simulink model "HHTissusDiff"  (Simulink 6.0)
settings: Solver=ode45  StartTime=0.0  StopTime=100  RelTol=1e-3
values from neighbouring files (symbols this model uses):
  b = S/Sm    (= 0.1)    [Constantes.m]    (also in ConstantesBck.m)
  C = 1    [Constantes.m]    (also in ConstantesBck.m)
  gk = 36    [Constantes.m]    (also in ConstantesBck.m; sim_hh.m)
  gl = 0.3    [Constantes.m]    (also in ConstantesBck.m; sim_hh.m)
  gna = 120    [Constantes.m]    (also in ConstantesBck.m; sim_hh.m)
  h0 = 0.5961    [Constantes.m]    (also in ConstantesBck.m)
  m0 = 0.0529    [Constantes.m]    (also in ConstantesBck.m)
  mK = 0    [Constantes.m]    (also in ConstantesBck.m)
  mL = 0    [Constantes.m]    (also in ConstantesBck.m)
  mNa = 0    [Constantes.m]    (also in ConstantesBck.m)
  n0 = 0.3177    [Constantes.m]    (also in ConstantesBck.m)
  Rext = 2.9E3    (= 2900)    [Constantes.m]    (also in ConstantesBck.m)
  Rint = 2.9E2    (= 290)    [Constantes.m]    (also in ConstantesBck.m = 400)
  Sm = 3.14e-2    (= 0.0314)    [Constantes.m]    (also in ConstantesBck.m = 0.000314)
  Vdd = 3.3*Rcan/Rct*1000    (= 3.2147881681)    [Constantes.m]    (also in ConstantesBck.m = 1.8)
  Vk = -82    [Constantes.m]    (also in ConstantesBck.m)
  Vl = -59    [Constantes.m]    (also in ConstantesBck.m)
  Vna = 45    [Constantes.m]    (also in ConstantesBck.m)
  Vr = -70    [Constantes.m]    (also in ConstantesBck.m)
libraries: simulink x2

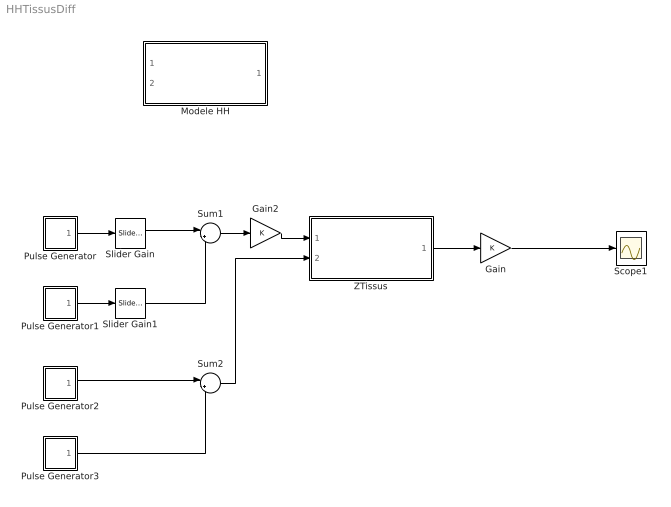
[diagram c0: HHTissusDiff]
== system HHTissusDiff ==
  Gain : Gain
  Gain2 : Gain
  Modele HH : Subsystem
  Pulse Generator : Subsystem  mask(Pulse Generator){period=50, duty=4, amplitude=-1E-2, start=10}
      mask prompts: period "Period (secs):"; duty "Duty cycle (% of period):"; start "Start time:"
      mask help: Pulse Generator
  Pulse Generator1 : Subsystem  mask(Pulse Generator){period=50, duty=4, amplitude=1E-2, start=12}
      mask prompts: period "Period (secs):"; duty "Duty cycle (% of period):"; start "Start time:"
      mask help: Pulse Generator
  Pulse Generator2 : Subsystem  mask(Pulse Generator){period=50, duty=4, amplitude=Vdd, start=10}
      mask prompts: period "Period (secs):"; duty "Duty cycle (% of period):"; start "Start time:"
      mask help: Pulse Generator
  Pulse Generator3 : Subsystem  mask(Pulse Generator){period=50, duty=4, amplitude=-Vdd, start=14}
      mask prompts: period "Period (secs):"; duty "Duty cycle (% of period):"; start "Start time:"
      mask help: Pulse Generator
  Scope1 : Scope
  Slider Gain : simulink/Math Operations/Slider Gain  low=0  gain=11  high=100
  Slider Gain1 : simulink/Math Operations/Slider Gain  low=0  gain=11  high=100
  Sum1 : Sum  Inputs=|++
  Sum2 : Sum  Inputs=|++
  ZTissus : Subsystem
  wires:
  ZTissus/1(Vout) -> Gain/1
  Pulse Generator/1(out1) -> Slider Gain/1
  Pulse Generator1/1(out1) -> Slider Gain1/1
  Slider Gain/1 -> Sum1/1
  Gain/1 -> Scope1/1
  Pulse Generator2/1(out1) -> Sum2/1
  Pulse Generator3/1(out1) -> Sum2/2
  Sum1/1 -> Gain2/1
  Gain2/1 -> ZTissus/1(IStim)
  Sum2/1 -> ZTissus/2(Vref)
  Slider Gain1/1 -> Sum1/2

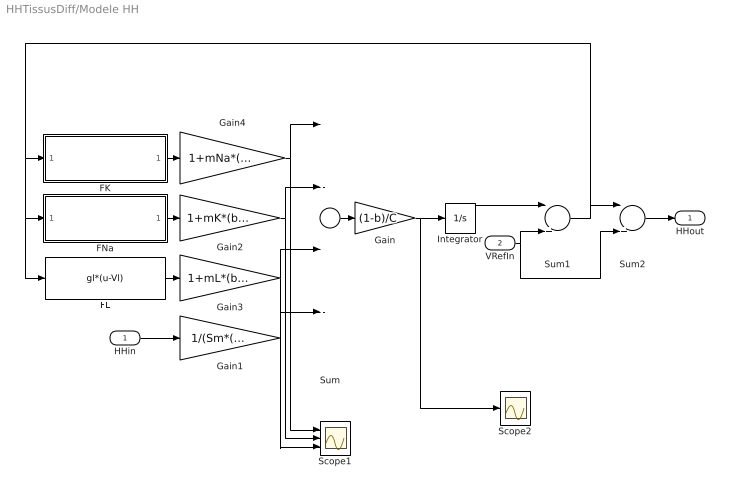
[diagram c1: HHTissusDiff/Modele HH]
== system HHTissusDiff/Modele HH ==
  HHin : Inport  Port=1  LatchInput=off
  VRefIn : Inport  Port=2  LatchInput=off
  FK : Subsystem
  FL : Fcn  Expr=gl*(u-Vl)
  FNa : Subsystem
  Gain : Gain  Gain=(1-b)/C
  Gain1 : Gain  Gain=1/(Sm*(1-b))
  Gain2 : Gain  Gain=1+mK*(b/(1-b))
  Gain3 : Gain  Gain=1+mL*(b/(1-b))
  Gain4 : Gain  Gain=1+mNa*(b/(1-b))
  Integrator : Integrator  InitialCondition=Vr
  Scope1 : Scope  NumInputPorts=3
  Scope2 : Scope
  Sum : Sum  Inputs=|---+
  Sum1 : Sum  Inputs=|++
  Sum2 : Sum  Inputs=|+-
  HHout : Outport
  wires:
  Sum/1 -> Gain/1
  Gain/1 -> Integrator/1, Scope2/1
  FK/1(FKout) -> Gain4/1
  FNa/1(FNaOut) -> Gain2/1
  FL/1 -> Gain3/1
  HHin/1 -> Gain1/1
  Integrator/1 -> Sum1/1
  Sum1/1 -> FNa/1(FNaIn), FL/1, FK/1(FKIn), Sum2/1
  VRefIn/1 -> Sum1/2, Sum2/2
  Gain1/1 -> Sum/4
  Gain4/1 -> Sum/1, Scope1/1
  Gain2/1 -> Sum/2, Scope1/2
  Gain3/1 -> Sum/3, Scope1/3
  Sum2/1 -> HHout/1

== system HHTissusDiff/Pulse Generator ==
  Constant1 : Constant  Value=0
  Sine Wave : Sin  Frequency=2*pi./period  Phase=-2*pi*(start./period + duty/200 - 1/4)
  Step : Step  Time=start  After=amplitude
  Switch : Switch  Threshold=sin(pi*(0.5 - duty/100))
  out1 : Outport  InitialOutput=0
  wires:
  Step/1 -> Switch/1
  Constant1/1 -> Switch/3
  Switch/1 -> out1/1
  Sine Wave/1 -> Switch/2

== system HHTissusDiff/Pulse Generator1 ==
  Constant1 : Constant  Value=0
  Sine Wave : Sin  Frequency=2*pi./period  Phase=-2*pi*(start./period + duty/200 - 1/4)
  Step : Step  Time=start  After=amplitude
  Switch : Switch  Threshold=sin(pi*(0.5 - duty/100))
  out1 : Outport  InitialOutput=0
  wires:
  Step/1 -> Switch/1
  Constant1/1 -> Switch/3
  Switch/1 -> out1/1
  Sine Wave/1 -> Switch/2

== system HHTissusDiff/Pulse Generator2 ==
  Constant1 : Constant  Value=0
  Sine Wave : Sin  Frequency=2*pi./period  Phase=-2*pi*(start./period + duty/200 - 1/4)
  Step : Step  Time=start  After=amplitude
  Switch : Switch  Threshold=sin(pi*(0.5 - duty/100))
  out1 : Outport  InitialOutput=0
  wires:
  Step/1 -> Switch/1
  Constant1/1 -> Switch/3
  Switch/1 -> out1/1
  Sine Wave/1 -> Switch/2

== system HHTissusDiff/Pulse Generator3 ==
  Constant1 : Constant  Value=0
  Sine Wave : Sin  Frequency=2*pi./period  Phase=-2*pi*(start./period + duty/200 - 1/4)
  Step : Step  Time=start  After=amplitude
  Switch : Switch  Threshold=sin(pi*(0.5 - duty/100))
  out1 : Outport  InitialOutput=0
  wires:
  Step/1 -> Switch/1
  Constant1/1 -> Switch/3
  Switch/1 -> out1/1
  Sine Wave/1 -> Switch/2

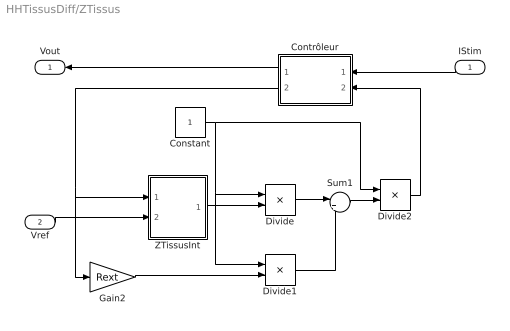
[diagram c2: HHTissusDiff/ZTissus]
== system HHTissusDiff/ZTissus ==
  IStim : Inport  Orientation=left  Port=1  LatchInput=off
  Vref : Inport  Port=2  LatchInput=off
  Constant : Constant
  Contrôleur : Stateflow chart  Orientation=left
  Divide : Product  Inputs=*/  OutScaling=2^-10
  Divide1 : Product  Inputs=*/  OutScaling=2^-10
  Divide2 : Product  Inputs=*/  OutScaling=2^-10
  Gain2 : Gain  Gain=Rext
  Sum1 : Sum  Inputs=|++
  ZTissusInt : Subsystem
  Vout : Outport  Orientation=left
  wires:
  Constant/1 -> Divide/1, Divide1/1, Divide2/1
  ZTissusInt/1(Vout) -> Divide/2
  Gain2/1 -> Divide1/2
  Divide/1 -> Sum1/1
  Divide1/1 -> Sum1/2
  Sum1/1 -> Divide2/2
  Vref/1 -> ZTissusInt/2(VRefIn)
  Divide2/1 -> Contrôleur/2(calc)
  Contrôleur/2(temp) -> ZTissusInt/1(InStim), Gain2/1
  IStim/1 -> Contrôleur/1(u)
  Contrôleur/1(y) -> Vout/1

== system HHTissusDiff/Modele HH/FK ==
  note: gkm
  note: (Vm-Vk0)
  FKIn : Inport  Port=1  LatchInput=off
  (Vm-Vk0) : Fcn  Expr=(u-Vk)
  Product : Product
  n(Vm) : Subsystem
  n^4 : Fcn  Expr=gk*(u^4)
  FKout : Outport  InitialOutput=0
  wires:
  n(Vm)/1(n) -> n^4/1
  (Vm-Vk0)/1 -> Product/2
  Product/1 -> FKout/1
  n^4/1 -> Product/1
  FKIn/1 -> n(Vm)/1(Vm), (Vm-Vk0)/1

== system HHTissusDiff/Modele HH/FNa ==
  note: gNa*m^3
  note: m
  note: h
  note: gNam
  note: (Vm-VNa0)
  FNaIn : Inport  Port=1  LatchInput=off
  (Vm-VNa0) : Fcn  Expr=(u-Vna)
  Product : Product
  Product1 : Product
  gna*m^3 : Fcn  Expr=gna*u^3
  h(Vm) : Subsystem
  m(Vm) : Subsystem
  FNaOut : Outport  InitialOutput=0
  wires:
  (Vm-VNa0)/1 -> Product1/2
  gna*m^3/1 -> Product/1
  Product1/1 -> FNaOut/1
  FNaIn/1 -> m(Vm)/1(Vm), h(Vm)/1(Vm), (Vm-VNa0)/1
  m(Vm)/1(n) -> gna*m^3/1
  h(Vm)/1(h) -> Product/2
  Product/1 -> Product1/1

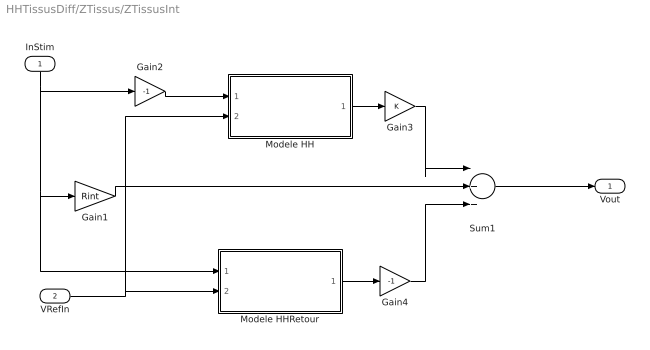
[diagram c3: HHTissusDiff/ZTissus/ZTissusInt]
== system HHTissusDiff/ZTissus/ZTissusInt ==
  InStim : Inport  Orientation=down  Port=1  LatchInput=off
  VRefIn : Inport  Port=2  LatchInput=off
  Gain1 : Gain  Gain=Rint
  Gain2 : Gain  Gain=-1
  Gain3 : Gain
  Gain4 : Gain  Gain=-1
  Modele HH : Subsystem
  Modele HHRetour : Subsystem
  Sum1 : Sum  Inputs=|+++
  Vout : Outport
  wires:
  Modele HH/1(HHout) -> Gain3/1
  Modele HHRetour/1(HHout) -> Gain4/1
  Gain1/1 -> Sum1/2
  InStim/1 -> Gain1/1, Modele HHRetour/1(HHin), Gain2/1
  Sum1/1 -> Vout/1
  VRefIn/1 -> Modele HHRetour/2(VRefIn), Modele HH/2(VRefIn)
  Gain3/1 -> Sum1/1
  Gain4/1 -> Sum1/3
  Gain2/1 -> Modele HH/1(HHin)

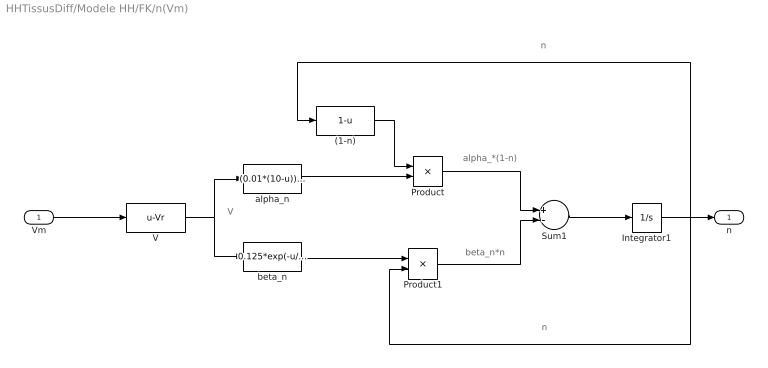
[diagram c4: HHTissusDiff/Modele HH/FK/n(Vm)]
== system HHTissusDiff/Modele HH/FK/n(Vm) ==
  note: V
  note: alpha_*(1-n)
  note: beta_n*n
  note: n
  note: n
  Vm : Inport  Port=1  LatchInput=off
  (1-n) : Fcn  Expr=1-u
  Integrator1 : Integrator  InitialCondition=n0
  Product : Product
  Product1 : Product
  Sum1 : Sum  Inputs=+-
  V : Fcn  Expr=u-Vr
  alpha_n : Fcn  Expr=(0.01*(10-u))/(exp((10-u)/10)-1)
  beta_n : Fcn  Expr=0.125*exp(-u/80)
  n : Outport  InitialOutput=0
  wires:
  V/1 -> alpha_n/1, beta_n/1
  alpha_n/1 -> Product/2
  (1-n)/1 -> Product/1
  beta_n/1 -> Product1/1
  Product/1 -> Sum1/1
  Product1/1 -> Sum1/2
  Sum1/1 -> Integrator1/1
  Integrator1/1 -> (1-n)/1, Product1/2, n/1
  Vm/1 -> V/1

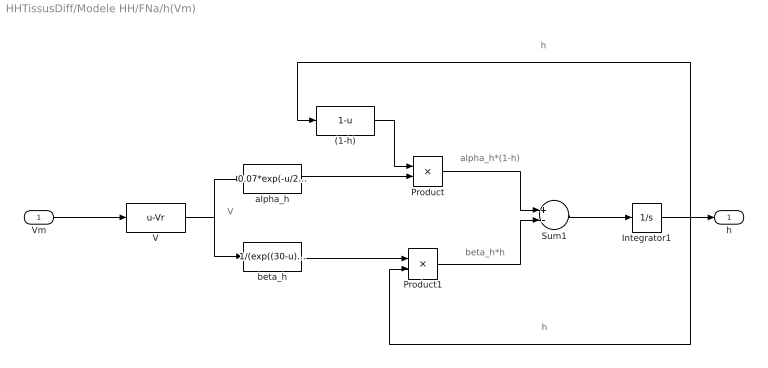
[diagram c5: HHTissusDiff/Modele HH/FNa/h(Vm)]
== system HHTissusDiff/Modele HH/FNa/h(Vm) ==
  note: h
  note: h
  note: beta_h*h
  note: alpha_h*(1-h)
  note: V
  Vm : Inport  Port=1  LatchInput=off
  (1-h) : Fcn  Expr=1-u
  Integrator1 : Integrator  InitialCondition=h0
  Product : Product
  Product1 : Product
  Sum1 : Sum  Inputs=+-
  V : Fcn  Expr=u-Vr
  alpha_h : Fcn  Expr=0.07*exp(-u/20)
  beta_h : Fcn  Expr=1/(exp((30-u)/10)+1)
  h : Outport  InitialOutput=0
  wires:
  Vm/1 -> V/1
  Integrator1/1 -> h/1, Product1/2, (1-h)/1
  Sum1/1 -> Integrator1/1
  Product1/1 -> Sum1/2
  Product/1 -> Sum1/1
  beta_h/1 -> Product1/1
  (1-h)/1 -> Product/1
  alpha_h/1 -> Product/2
  V/1 -> beta_h/1, alpha_h/1

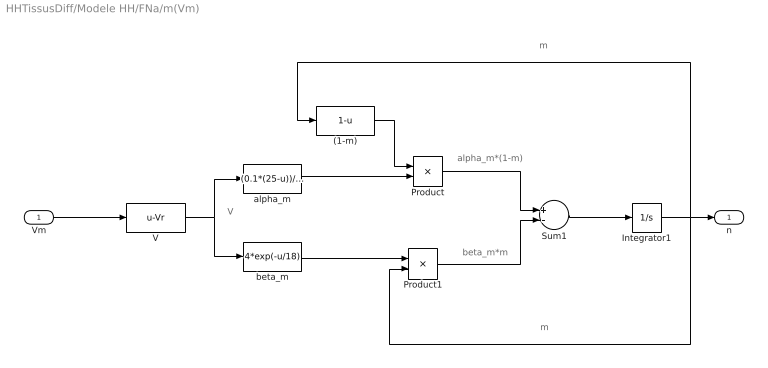
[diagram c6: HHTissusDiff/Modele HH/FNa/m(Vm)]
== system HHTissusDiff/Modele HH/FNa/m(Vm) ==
  note: m
  note: m
  note: beta_m*m
  note: alpha_m*(1-m)
  note: V
  Vm : Inport  Port=1  LatchInput=off
  (1-m) : Fcn  Expr=1-u
  Integrator1 : Integrator  InitialCondition=m0
  Product : Product
  Product1 : Product
  Sum1 : Sum  Inputs=+-
  V : Fcn  Expr=u-Vr
  alpha_m : Fcn  Expr=(0.1*(25-u))/(exp((25-u)/10)-1)
  beta_m : Fcn  Expr=4*exp(-u/18)
  n : Outport  InitialOutput=0
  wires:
  Vm/1 -> V/1
  Integrator1/1 -> n/1, Product1/2, (1-m)/1
  Sum1/1 -> Integrator1/1
  Product1/1 -> Sum1/2
  Product/1 -> Sum1/1
  beta_m/1 -> Product1/1
  (1-m)/1 -> Product/1
  alpha_m/1 -> Product/2
  V/1 -> beta_m/1, alpha_m/1

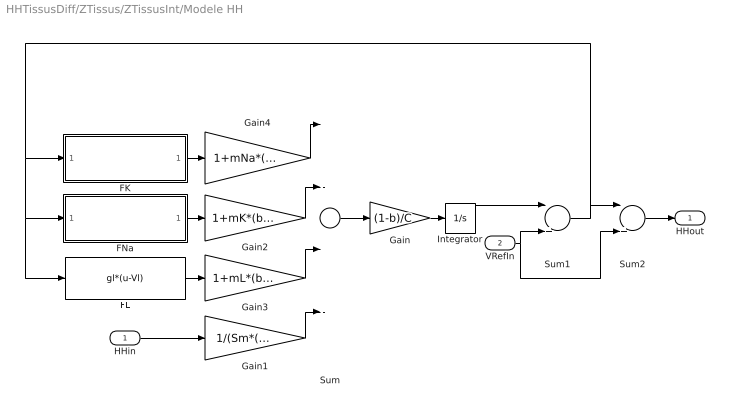
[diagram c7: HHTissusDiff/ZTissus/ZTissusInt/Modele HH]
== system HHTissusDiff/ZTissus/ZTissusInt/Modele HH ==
  HHin : Inport  Port=1  LatchInput=off
  VRefIn : Inport  Port=2  LatchInput=off
  FK : Subsystem
  FL : Fcn  Expr=gl*(u-Vl)
  FNa : Subsystem
  Gain : Gain  Gain=(1-b)/C
  Gain1 : Gain  Gain=1/(Sm*(1-b))
  Gain2 : Gain  Gain=1+mK*(b/(1-b))
  Gain3 : Gain  Gain=1+mL*(b/(1-b))
  Gain4 : Gain  Gain=1+mNa*(b/(1-b))
  Integrator : Integrator  InitialCondition=Vr
  Sum : Sum  Inputs=|---+
  Sum1 : Sum  Inputs=|++
  Sum2 : Sum  Inputs=|+-
  HHout : Outport
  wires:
  Sum/1 -> Gain/1
  Gain/1 -> Integrator/1
  FK/1(FKout) -> Gain4/1
  FNa/1(FNaOut) -> Gain2/1
  FL/1 -> Gain3/1
  HHin/1 -> Gain1/1
  Integrator/1 -> Sum1/1
  Sum1/1 -> FNa/1(FNaIn), FL/1, FK/1(FKIn), Sum2/1
  VRefIn/1 -> Sum1/2, Sum2/2
  Gain1/1 -> Sum/4
  Gain4/1 -> Sum/1
  Gain2/1 -> Sum/2
  Gain3/1 -> Sum/3
  Sum2/1 -> HHout/1

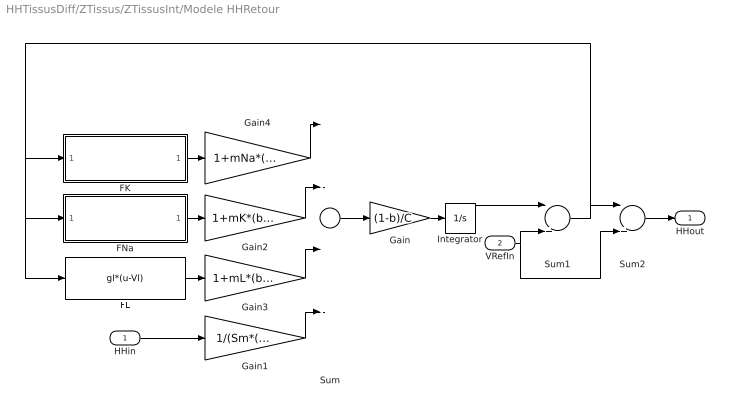
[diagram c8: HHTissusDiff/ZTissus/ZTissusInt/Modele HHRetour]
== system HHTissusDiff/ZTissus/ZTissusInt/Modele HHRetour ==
  HHin : Inport  Port=1  LatchInput=off
  VRefIn : Inport  Port=2  LatchInput=off
  FK : Subsystem
  FL : Fcn  Expr=gl*(u-Vl)
  FNa : Subsystem
  Gain : Gain  Gain=(1-b)/C
  Gain1 : Gain  Gain=1/(Sm*(1-b))
  Gain2 : Gain  Gain=1+mK*(b/(1-b))
  Gain3 : Gain  Gain=1+mL*(b/(1-b))
  Gain4 : Gain  Gain=1+mNa*(b/(1-b))
  Integrator : Integrator  InitialCondition=Vr
  Sum : Sum  Inputs=|---+
  Sum1 : Sum  Inputs=|++
  Sum2 : Sum  Inputs=|+-
  HHout : Outport
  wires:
  Sum/1 -> Gain/1
  Gain/1 -> Integrator/1
  FK/1(FKout) -> Gain4/1
  FNa/1(FNaOut) -> Gain2/1
  FL/1 -> Gain3/1
  HHin/1 -> Gain1/1
  Integrator/1 -> Sum1/1
  Sum1/1 -> FNa/1(FNaIn), FL/1, FK/1(FKIn), Sum2/1
  VRefIn/1 -> Sum1/2, Sum2/2
  Gain1/1 -> Sum/4
  Gain4/1 -> Sum/1
  Gain2/1 -> Sum/2
  Gain3/1 -> Sum/3
  Sum2/1 -> HHout/1

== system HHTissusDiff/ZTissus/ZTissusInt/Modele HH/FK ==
  note: gkm
  note: (Vm-Vk0)
  FKIn : Inport  Port=1  LatchInput=off
  (Vm-Vk0) : Fcn  Expr=(u-Vk)
  Product : Product
  n(Vm) : Subsystem
  n^4 : Fcn  Expr=gk*(u^4)
  FKout : Outport  InitialOutput=0
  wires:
  n(Vm)/1(n) -> n^4/1
  (Vm-Vk0)/1 -> Product/2
  Product/1 -> FKout/1
  n^4/1 -> Product/1
  FKIn/1 -> n(Vm)/1(Vm), (Vm-Vk0)/1

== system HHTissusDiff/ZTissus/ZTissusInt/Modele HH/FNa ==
  note: gNa*m^3
  note: m
  note: h
  note: gNam
  note: (Vm-VNa0)
  FNaIn : Inport  Port=1  LatchInput=off
  (Vm-VNa0) : Fcn  Expr=(u-Vna)
  Product : Product
  Product1 : Product
  gna*m^3 : Fcn  Expr=gna*u^3
  h(Vm) : Subsystem
  m(Vm) : Subsystem
  FNaOut : Outport  InitialOutput=0
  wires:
  (Vm-VNa0)/1 -> Product1/2
  gna*m^3/1 -> Product/1
  Product1/1 -> FNaOut/1
  FNaIn/1 -> m(Vm)/1(Vm), h(Vm)/1(Vm), (Vm-VNa0)/1
  m(Vm)/1(n) -> gna*m^3/1
  h(Vm)/1(h) -> Product/2
  Product/1 -> Product1/1

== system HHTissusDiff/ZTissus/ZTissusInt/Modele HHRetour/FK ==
  note: gkm
  note: (Vm-Vk0)
  FKIn : Inport  Port=1  LatchInput=off
  (Vm-Vk0) : Fcn  Expr=(u-Vk)
  Product : Product
  n(Vm) : Subsystem
  n^4 : Fcn  Expr=gk*(u^4)
  FKout : Outport  InitialOutput=0
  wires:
  n(Vm)/1(n) -> n^4/1
  (Vm-Vk0)/1 -> Product/2
  Product/1 -> FKout/1
  n^4/1 -> Product/1
  FKIn/1 -> n(Vm)/1(Vm), (Vm-Vk0)/1

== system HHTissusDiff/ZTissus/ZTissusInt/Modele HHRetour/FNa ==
  note: gNa*m^3
  note: m
  note: h
  note: gNam
  note: (Vm-VNa0)
  FNaIn : Inport  Port=1  LatchInput=off
  (Vm-VNa0) : Fcn  Expr=(u-Vna)
  Product : Product
  Product1 : Product
  gna*m^3 : Fcn  Expr=gna*u^3
  h(Vm) : Subsystem
  m(Vm) : Subsystem
  FNaOut : Outport  InitialOutput=0
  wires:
  (Vm-VNa0)/1 -> Product1/2
  gna*m^3/1 -> Product/1
  Product1/1 -> FNaOut/1
  FNaIn/1 -> m(Vm)/1(Vm), h(Vm)/1(Vm), (Vm-VNa0)/1
  m(Vm)/1(n) -> gna*m^3/1
  h(Vm)/1(h) -> Product/2
  Product/1 -> Product1/1

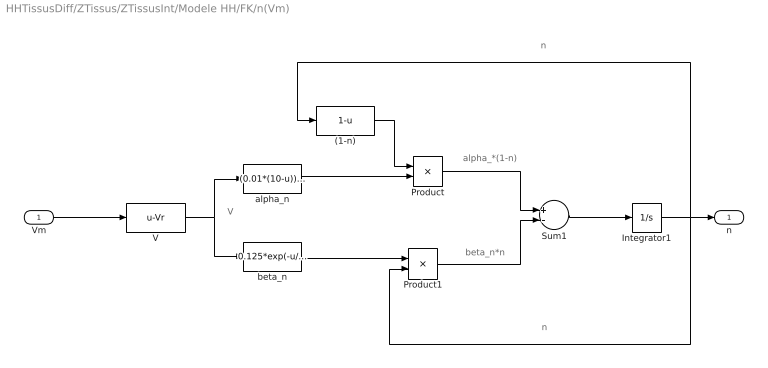
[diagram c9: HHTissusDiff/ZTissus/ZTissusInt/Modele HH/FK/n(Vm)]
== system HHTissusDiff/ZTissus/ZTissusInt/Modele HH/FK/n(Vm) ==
  note: V
  note: alpha_*(1-n)
  note: beta_n*n
  note: n
  note: n
  Vm : Inport  Port=1  LatchInput=off
  (1-n) : Fcn  Expr=1-u
  Integrator1 : Integrator  InitialCondition=n0
  Product : Product
  Product1 : Product
  Sum1 : Sum  Inputs=+-
  V : Fcn  Expr=u-Vr
  alpha_n : Fcn  Expr=(0.01*(10-u))/(exp((10-u)/10)-1)
  beta_n : Fcn  Expr=0.125*exp(-u/80)
  n : Outport  InitialOutput=0
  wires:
  V/1 -> alpha_n/1, beta_n/1
  alpha_n/1 -> Product/2
  (1-n)/1 -> Product/1
  beta_n/1 -> Product1/1
  Product/1 -> Sum1/1
  Product1/1 -> Sum1/2
  Sum1/1 -> Integrator1/1
  Integrator1/1 -> (1-n)/1, Product1/2, n/1
  Vm/1 -> V/1

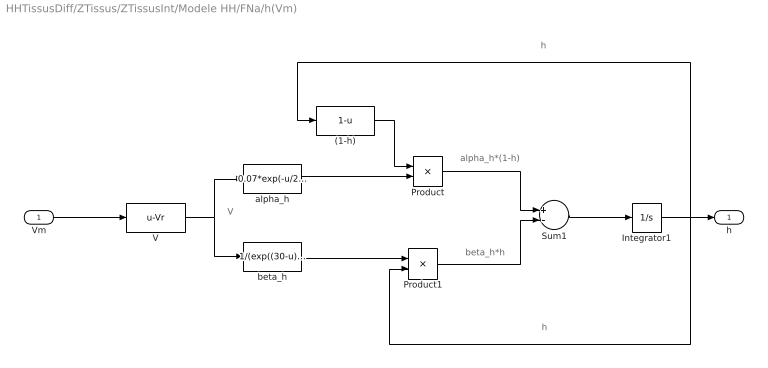
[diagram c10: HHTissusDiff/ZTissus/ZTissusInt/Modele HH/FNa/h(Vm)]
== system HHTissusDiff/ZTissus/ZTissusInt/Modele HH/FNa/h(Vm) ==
  note: h
  note: h
  note: beta_h*h
  note: alpha_h*(1-h)
  note: V
  Vm : Inport  Port=1  LatchInput=off
  (1-h) : Fcn  Expr=1-u
  Integrator1 : Integrator  InitialCondition=h0
  Product : Product
  Product1 : Product
  Sum1 : Sum  Inputs=+-
  V : Fcn  Expr=u-Vr
  alpha_h : Fcn  Expr=0.07*exp(-u/20)
  beta_h : Fcn  Expr=1/(exp((30-u)/10)+1)
  h : Outport  InitialOutput=0
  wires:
  Vm/1 -> V/1
  Integrator1/1 -> h/1, Product1/2, (1-h)/1
  Sum1/1 -> Integrator1/1
  Product1/1 -> Sum1/2
  Product/1 -> Sum1/1
  beta_h/1 -> Product1/1
  (1-h)/1 -> Product/1
  alpha_h/1 -> Product/2
  V/1 -> beta_h/1, alpha_h/1

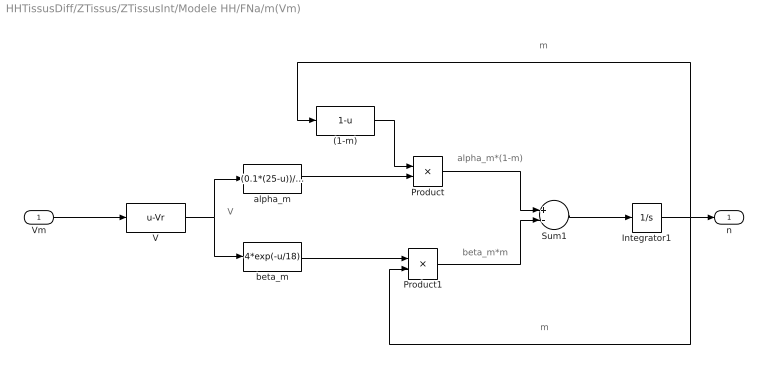
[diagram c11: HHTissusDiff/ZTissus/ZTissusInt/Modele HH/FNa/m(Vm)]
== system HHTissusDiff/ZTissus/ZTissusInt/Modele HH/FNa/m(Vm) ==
  note: m
  note: m
  note: beta_m*m
  note: alpha_m*(1-m)
  note: V
  Vm : Inport  Port=1  LatchInput=off
  (1-m) : Fcn  Expr=1-u
  Integrator1 : Integrator  InitialCondition=m0
  Product : Product
  Product1 : Product
  Sum1 : Sum  Inputs=+-
  V : Fcn  Expr=u-Vr
  alpha_m : Fcn  Expr=(0.1*(25-u))/(exp((25-u)/10)-1)
  beta_m : Fcn  Expr=4*exp(-u/18)
  n : Outport  InitialOutput=0
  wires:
  Vm/1 -> V/1
  Integrator1/1 -> n/1, Product1/2, (1-m)/1
  Sum1/1 -> Integrator1/1
  Product1/1 -> Sum1/2
  Product/1 -> Sum1/1
  beta_m/1 -> Product1/1
  (1-m)/1 -> Product/1
  alpha_m/1 -> Product/2
  V/1 -> beta_m/1, alpha_m/1

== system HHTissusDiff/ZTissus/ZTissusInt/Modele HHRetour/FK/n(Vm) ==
  note: V
  note: alpha_*(1-n)
  note: beta_n*n
  note: n
  note: n
  Vm : Inport  Port=1  LatchInput=off
  (1-n) : Fcn  Expr=1-u
  Integrator1 : Integrator  InitialCondition=n0
  Product : Product
  Product1 : Product
  Sum1 : Sum  Inputs=+-
  V : Fcn  Expr=u-Vr
  alpha_n : Fcn  Expr=(0.01*(10-u))/(exp((10-u)/10)-1)
  beta_n : Fcn  Expr=0.125*exp(-u/80)
  n : Outport  InitialOutput=0
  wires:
  V/1 -> alpha_n/1, beta_n/1
  alpha_n/1 -> Product/2
  (1-n)/1 -> Product/1
  beta_n/1 -> Product1/1
  Product/1 -> Sum1/1
  Product1/1 -> Sum1/2
  Sum1/1 -> Integrator1/1
  Integrator1/1 -> (1-n)/1, Product1/2, n/1
  Vm/1 -> V/1

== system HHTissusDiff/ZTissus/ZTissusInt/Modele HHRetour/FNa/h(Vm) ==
  note: h
  note: h
  note: beta_h*h
  note: alpha_h*(1-h)
  note: V
  Vm : Inport  Port=1  LatchInput=off
  (1-h) : Fcn  Expr=1-u
  Integrator1 : Integrator  InitialCondition=h0
  Product : Product
  Product1 : Product
  Sum1 : Sum  Inputs=+-
  V : Fcn  Expr=u-Vr
  alpha_h : Fcn  Expr=0.07*exp(-u/20)
  beta_h : Fcn  Expr=1/(exp((30-u)/10)+1)
  h : Outport  InitialOutput=0
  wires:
  Vm/1 -> V/1
  Integrator1/1 -> h/1, Product1/2, (1-h)/1
  Sum1/1 -> Integrator1/1
  Product1/1 -> Sum1/2
  Product/1 -> Sum1/1
  beta_h/1 -> Product1/1
  (1-h)/1 -> Product/1
  alpha_h/1 -> Product/2
  V/1 -> beta_h/1, alpha_h/1

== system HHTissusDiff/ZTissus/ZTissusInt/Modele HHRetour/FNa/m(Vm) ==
  note: m
  note: m
  note: beta_m*m
  note: alpha_m*(1-m)
  note: V
  Vm : Inport  Port=1  LatchInput=off
  (1-m) : Fcn  Expr=1-u
  Integrator1 : Integrator  InitialCondition=m0
  Product : Product
  Product1 : Product
  Sum1 : Sum  Inputs=+-
  V : Fcn  Expr=u-Vr
  alpha_m : Fcn  Expr=(0.1*(25-u))/(exp((25-u)/10)-1)
  beta_m : Fcn  Expr=4*exp(-u/18)
  n : Outport  InitialOutput=0
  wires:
  Vm/1 -> V/1
  Integrator1/1 -> n/1, Product1/2, (1-m)/1
  Sum1/1 -> Integrator1/1
  Product1/1 -> Sum1/2
  Product/1 -> Sum1/1
  beta_m/1 -> Product1/1
  (1-m)/1 -> Product/1
  alpha_m/1 -> Product/2
  V/1 -> beta_m/1, alpha_m/1

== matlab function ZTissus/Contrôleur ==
function [y,temp] = fcn(u,calc)
% This block supports an embeddable subset of the MATLAB language.
% See the help menu for details. 

if u == 0
    y = 0;
    temp = 1E-6;
else
    y = calc;
    temp = u;
end
